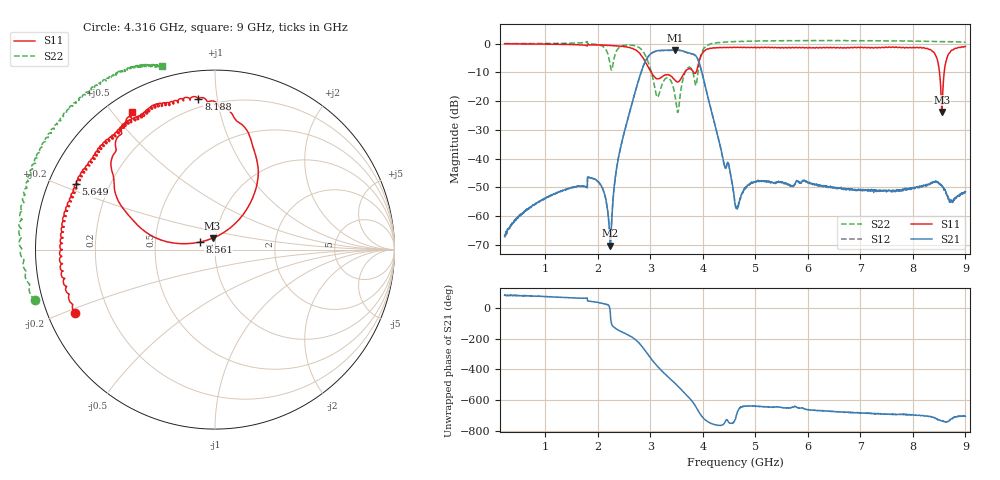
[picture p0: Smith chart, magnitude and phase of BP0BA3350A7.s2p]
!Agilent Technologies,E8358A,US41080443,A.07.50.56
!Agilent E8358A: A.07.50.56
!Date: Friday, July 21, 2017 20:21:57
!Correction: S11(Full 2 Port(1,2))
!S21(Full 2 Port(1,2))
!S12(Full 2 Port(1,2))
!S22(Full 2 Port(1,2))
!S2P File: Measurements: S11, S21, S12, S22:
# Hz S  dB  R 50
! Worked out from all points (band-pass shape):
!   1601 points, 225 MHz to 9 GHz, reference 50 ohm
!   highest |S21| = -2.17 dB at 3.477 GHz (marker M1); lowest = -70.3 dB at 2.238 GHz (marker M2)
!   |S21| within 3 dB of the highest: 2.934 GHz to 3.899 GHz (964.7 MHz wide, 28.2 % of centre)
!   lowest |S11| = -23.8 dB at 8.55 GHz (marker M3), VSWR 1.14, Z = 48.3 + j6.15 ohm
!   |S11| at or under -10 dB: 3.017 GHz to 3.652 GHz (635.1 MHz wide, 19 % of centre); 3.825 GHz to 3.87 GHz (45.3 MHz wide, 1.18 % of centre); 8.507 GHz to 8.596 GHz (89 MHz wide, 1.04 % of centre)
!   |S22| runs from -24.0 to 1.1 dB; largest |S21 - S12| = 0.013
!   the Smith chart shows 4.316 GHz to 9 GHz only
!   S11 on the Smith chart (normalised r, x): 4.316 GHz: 0.08, -0.21; 5.649 GHz: 0.08, +0.22; 8.188 GHz: 0.15, +0.89; 8.561 GHz: 0.84, +0.07; 9 GHz: 0.07, +0.56
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2.25e8  -0.05 177.4  -66.82 81.8  -67.44 80.7  0.02 176.3
1.689328e9  -0.44 147.0  -49.51 62.8  -49.60 62.9  0.32 160.2
2.062266e9  -0.50 141.8  -49.34 31.3  -49.47 30.8  -0.68 92.9
2.237766e9  -0.68 131.3  -70.25 -28.1  -70.42 -37.5  -7.61 -10.5
2.396812e9  -0.81 119.1  -39.23 -146.2  -39.35 -146.4  -1.53 161.1
2.649094e9  -1.61 79.8  -20.88 169.5  -21.02 169.3  -0.59 109.2
2.813625e9  -3.74 18.7  -10.52 119.9  -10.57 119.6  -1.75 75.3
2.967188e9  -8.42 -76.7  -4.27 49.9  -4.39 50.1  -6.75 32.0
3.153656e9  -12.22 -132.3  -2.39 -27.9  -2.50 -28.4  -18.22 -105.9
3.477234e9  -12.86 -150.8  -2.17 -134.3  -2.28 -134.8  -18.87 85.2
3.811781e9  -9.63 -135.6  -3.59 104.5  -3.71 104.1  -10.11 -154.5
4.025672e9  -2.59 -123.7  -13.28 -4.1  -13.36 -4.6  -1.49 -122.7
4.316344e9  -1.37 -155.7  -34.51 -45.8  -34.56 -46.7  0.34 -164.3
4.6125e9  -1.32 -171.9  -55.57 -10.0  -55.29 -11.2  0.76 177.6
5.649047e9  -1.33 154.9  -49.22 68.5  -49.37 67.7  1.06 145.6
6.076828e9  -1.50 144.9  -48.56 54.2  -48.66 52.7  1.03 136.0
7.541156e9  -1.18 114.0  -51.08 27.5  -51.15 27.8  0.92 115.4
8.188312e9  -1.45 96.3  -49.39 18.4  -49.46 17.2  0.79 110.9
8.550281e9  -23.77 102.0  -49.24 -17.3  -49.46 -18.0  0.73 109.3
8.56125e9  -20.41 154.1  -49.55 -16.5  -49.76 -17.7  0.75 109.0
8.687391e9  -3.42 146.5  -54.43 -17.6  -54.32 -16.9  0.70 108.6
9e9  -0.95 121.1  -51.50 13.8  -51.60 17.1  0.53 106.2
